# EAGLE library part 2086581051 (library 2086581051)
1.0 HDMI R/A HEADER ASSy (I/M type) Source: Datasheet
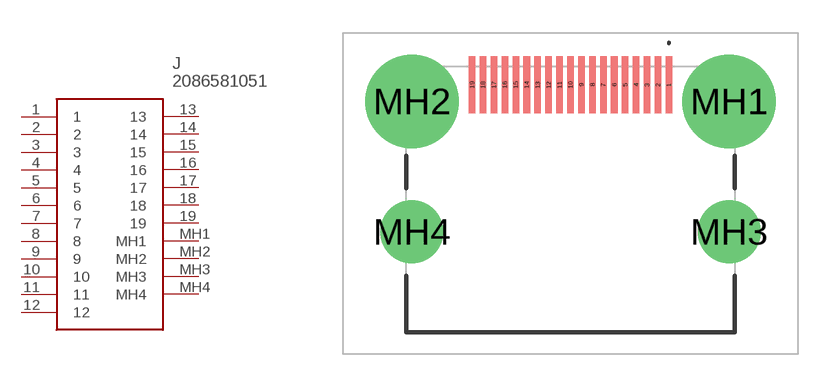
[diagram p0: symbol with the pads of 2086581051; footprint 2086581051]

Designator prefix J

## 2086581051 (Arrow_Part_Number: 2086581051; Arrow_Price-Stock: https://www.arrow.com/en/products/2086581051/molex?region=nac; Description: 1.0 HDMI R/A HEADER ASSy (I/M type); Height: 6.44mm; Manufacturer_Name: Molex; Manufacturer_Part_Number: 2086581051)  [2086581051]
1  1
2  2
3  3
4  4
5  5
6  6
7  7
8  8
9  9
10  10
11  11
12  12
13  13
14  14
15  15
16  16
17  17
18  18
19  19
MH1  MH1
MH2  MH2
MH3  MH3
MH4  MH4

## Footprint 2086581051 (pad centres in mm)
2086581051-1
smd 0.3 x 2.6: 1 4.5,5.235; 2 4,5.235; 3 3.5,5.235; 4 3,5.235; 5 2.5,5.235; 6 2,5.235; 7 1.5,5.235; 8 1,5.235; 9 0.5,5.235; 10 0,5.235; 11 -0.5,5.235; 12 -1,5.235; 13 -1.5,5.235; 14 -2,5.235; 15 -2.5,5.235; 16 -3,5.235; 17 -3.5,5.235; 18 -4,5.235; 19 -4.5,5.235
drill 2.85 pad 4.275: MH1 7.25,4.475; MH2 -7.25,4.475
drill 1.92 pad 2.88: MH3 7.25,-1.485; MH4 -7.25,-1.485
